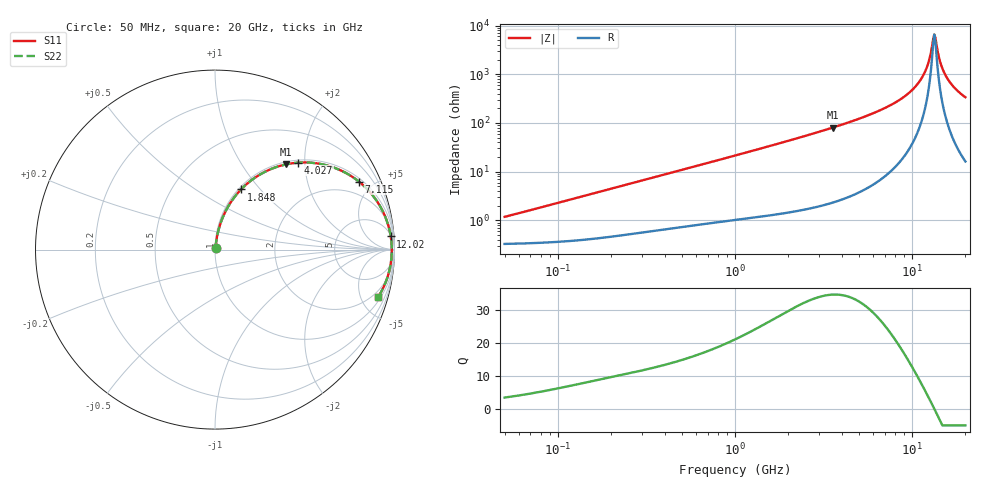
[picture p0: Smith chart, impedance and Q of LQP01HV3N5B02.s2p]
!Murata Part Number: LQP01HV3N5B02
!These Parameters are Measured in Series Mode Connection
!  o--[Z]--o
!Port1  Port2
!  o-------o
!Freq. Start=50[MHz] Stop=20[GHz], 401[Steps]
# Hz S RI R 50
!Freq.(Hz) S11(Real) S11(Imag) S21(Real) S21(Imag) S12(Real) S12(Imag) S22(Real) S22(Imag)
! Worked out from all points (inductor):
!   401 points, 50 MHz to 20 GHz, reference 50 ohm
!   read as one part in series: L = 3.62 nH near 51.52 MHz
!   highest Q = 34.6 at 3.572 GHz (marker M1), where L = 3.59 nH
!   self-resonance near 13.35 GHz
!   S11 on the Smith chart (normalised r, x): 50 MHz: 1.01, +0.02; 1.848 GHz: 1.03, +0.79; 4.027 GHz: 1.05, +1.86; 7.115 GHz: 1.17, +4.15; 12.02 GHz: 6, +25; 20 GHz: 1.32, -6.74
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5e7  0.00341 0.0113  0.9966 -0.0113  0.9966 -0.0113  0.00341 0.0113
1.364002e8  0.00489 0.0305  0.9951 -0.0305  0.9951 -0.0305  0.00489 0.0305
3.721004e8  0.0128 0.08  0.9872 -0.08  0.9872 -0.08  0.0128 0.08
1e9  0.0526 0.2008  0.9474 -0.2008  0.9474 -0.2008  0.0526 0.2008
1.848039e9  0.1448 0.335  0.8552 -0.335  0.8552 -0.335  0.1448 0.335
2.728004e9  0.2695 0.4289  0.7305 -0.4289  0.7305 -0.4289  0.2695 0.4289
3.572216e9  0.3971 0.4751  0.6029 -0.4751  0.6029 -0.4751  0.3971 0.4751
4.026975e9  0.4638 0.4844  0.5362 -0.4844  0.5362 -0.4844  0.4638 0.4844
5.352748e9  0.6362 0.4655  0.3638 -0.4655  0.3638 -0.4655  0.6362 0.4655
7.114996e9  0.8022 0.3787  0.1978 -0.3787  0.1978 -0.3787  0.8022 0.3787
7.442007e9  0.8254 0.3589  0.1746 -0.3589  0.1746 -0.3589  0.8254 0.3589
1.004137e10  0.9445 0.1927  0.0555 -0.1927  0.0555 -0.1927  0.9445 0.1927
1.115139e10  0.9684 0.1242  0.0316 -0.1242  0.0316 -0.1242  0.9684 0.1242
1.201863e10  0.9791 0.0734  0.0209 -0.0734  0.0209 -0.0734  0.9791 0.0734
1.238412e10  0.9819 0.0528  0.0181 -0.0528  0.0181 -0.0528  0.9819 0.0528
1.314879e10  0.9848 0.0114  0.0152 -0.0114  0.0152 -0.0114  0.9848 0.0114
1.334722e10  0.985 0.000995  0.015 -0.000995  0.015 -0.000995  0.985 0.000995
1.375312e10  0.9847 -0.0198  0.0153 0.0198  0.0153 0.0198  0.9847 -0.0198
1.460232e10  0.9815 -0.0613  0.0185 0.0613  0.0185 0.0613  0.9815 -0.0613
1.550395e10  0.9747 -0.1023  0.0253 0.1023  0.0253 0.1023  0.9747 -0.1023
1.721783e10  0.9546 -0.1723  0.0454 0.1723  0.0454 0.1723  0.9546 -0.1723
2e10  0.9084 -0.2653  0.0916 0.2653  0.0916 0.2653  0.9084 -0.2653
